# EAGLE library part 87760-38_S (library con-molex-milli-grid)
HEADER
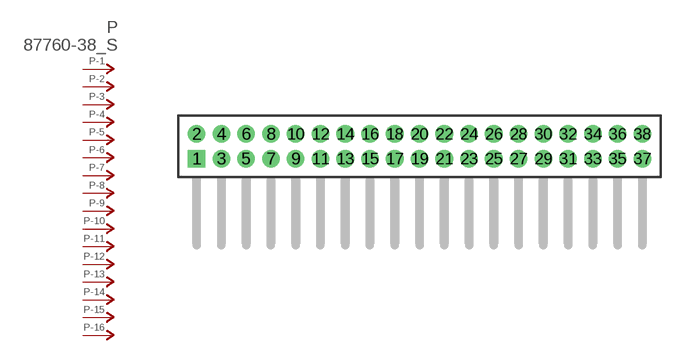
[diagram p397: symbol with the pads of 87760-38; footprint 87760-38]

Designator prefix P; gates -1=P-NV -2=P-N -3=P-N -4=P-N -5=P-N -6=P-N -7=P-N -8=P-N -9=P-N -10=P-N -11=P-N -12=P-N -13=P-N -14=P-N -15=P-N -16=P-N -17=P-N -18=P-N -19=P-N -20=P-N -21=P-N -22=P-N -23=P-N -24=P-N -25=P-N -26=P-N -27=P-N -28=P-N -29=P-N -30=P-N -31=P-N -32=P-N -33=P-N -34=P-N -35=P-N -36=P-N -37=P-N -38=P-N

## 87760-38_S  [87760-38]
1  -1:P  pas
2  -2:P  pas
3  -3:P  pas
4  -4:P  pas
5  -5:P  pas
6  -6:P  pas
7  -7:P  pas
8  -8:P  pas
9  -9:P  pas
10  -10:P  pas
11  -11:P  pas
12  -12:P  pas
13  -13:P  pas
14  -14:P  pas
15  -15:P  pas
16  -16:P  pas
17  -17:P  pas
18  -18:P  pas
19  -19:P  pas
20  -20:P  pas
21  -21:P  pas
22  -22:P  pas
23  -23:P  pas
24  -24:P  pas
25  -25:P  pas
26  -26:P  pas
27  -27:P  pas
28  -28:P  pas
29  -29:P  pas
30  -30:P  pas
31  -31:P  pas
32  -32:P  pas
33  -33:P  pas
34  -34:P  pas
35  -35:P  pas
36  -36:P  pas
37  -37:P  pas
38  -38:P  pas

## Footprint 87760-38 (pad centres in mm)
HEADER Dual Row, Right Angle
drill 0.914 square: 1 -18,-1
drill 0.914: 2 -18,1; 3 -16,-1; 4 -16,1; 5 -14,-1; 6 -14,1; 7 -12,-1; 8 -12,1; 9 -10,-1; 10 -10,1; 11 -8,-1; 12 -8,1; 13 -6,-1; 14 -6,1; 15 -4,-1; 16 -4,1; 17 -2,-1; 18 -2,1; 19 0,-1; 20 0,1; 21 2,-1; 22 2,1; 23 4,-1; 24 4,1; 25 6,-1; 26 6,1; 27 8,-1; 28 8,1; 29 10,-1; 30 10,1; 31 12,-1; 32 12,1; 33 14,-1; 34 14,1; 35 16,-1; 36 16,1; 37 18,-1; 38 18,1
